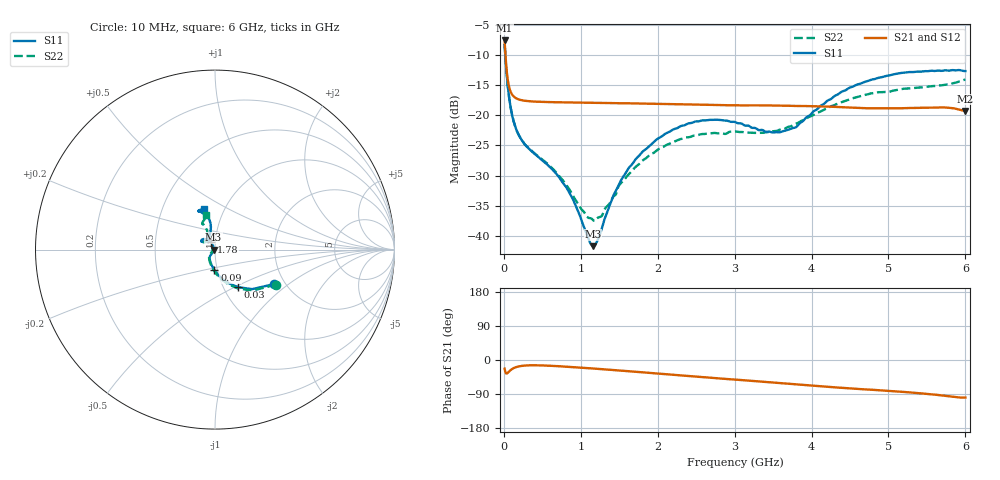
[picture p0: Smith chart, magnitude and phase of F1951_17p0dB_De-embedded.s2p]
! Integrated Device Technology
! Corporate Headquarters
! 6024 Silver Creek Valley Road
! San Jose, CA 95138  USA
! Phone:  1-408-284-8200
! Toll Free:  1-800-223-1366
! Webpage:  http://www.idt.com/
! Timing and RF Division
! 515 Groton Road, Suite 102
! Westford, MA 01886-6024
! Device:  F1951
! Description: 6-bit 0.5 dB Digital Step Attenuator
! Frequency:  100.0 -  4000.00 MHz
! Package:  4x4 mm Thin QFN Plastic Package: 24 pin
! Ports:  2 RF, 6 DC
!  Pin  1  = NC
!  Pin  2  = RF1  =  Port 1
!  Pin  3  = GND
!  Pin  4  = NC
!  Pin  5  = Serial Data Out (SDO)
!  Pin  6  = NC
!  Pin  7  = Reset Bar ( RSTb)
!  Pin  8  = Clock (CLK)
!  Pin  9  = Chip Select Bar (CSb)
!  Pin 10  = NC
!  Pin 11  = Serial Data In (SDI)
!  Pin 12  = NC
!  Pin 13  = NC
!  Pin 14  = VDD
!  Pin 15  = NC
!  Pin 16  = GND
!  Pin 17  = RF2  =  Port 2
!  Pin 18  = NC
!  Pin 19  = GND
!  Pin 20  = GND
!  Pin 21  = GND
!  Pin 22  = GND
!  Pin 23  = GND
!  Pin 24  = GND
! State:  34
! Atten State:  17.0 dB
! Voltage:  +3.30 Volts
! Current:  0.478 mA
! Data:  The device was measured on a F195X evaluation board which has
!  individual transmission lines to the RF pins.  Data was collected
!  de-embedded using a Automatic Fixture Removal [AFR] (Keysight Technologies).
!  The reference plane is the edge of the package pin.
! Misc:  Lot Code  1225BCA
!  Action Tracker AT0399
! Date Measured:  2018-09-13
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# GHz S dB R 50
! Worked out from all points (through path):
!   600 points, 10 MHz to 6 GHz, reference 50 ohm
!   highest |S21| = -7.60 dB at 10 MHz (marker M1); lowest = -19.3 dB at 6 GHz (marker M2)
!   group delay of S21, straight-line fit = 41 ps
!   lowest |S11| = -41.7 dB at 1.16 GHz (marker M3), VSWR 1.02, Z = 49.2 + j0.0511 ohm
!   |S11| at or under -10 dB: 18.05 MHz to end of sweep
!   |S22| runs from -37.5 to -8.2 dB; largest |S21 - S12| = 0.00027
!   S11 on the Smith chart (normalised r, x): 10 MHz: 1.76, -0.79; 30 MHz: 1.17, -0.52; 90 MHz: 0.97, -0.22; 1.78 GHz: 0.95, +0.08; 6 GHz: 0.80, +0.38
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0.01  -8.36 -30.2  -7.60 -23.0  -7.60 -23.0  -8.15 -30.0
0.03  -12.18 -58.3  -11.58 -35.5  -11.58 -35.6  -12.03 -59.7
0.06  -16.19 -79.2  -14.81 -32.1  -14.82 -32.1  -16.16 -81.2
0.09  -18.85 -91.4  -16.15 -26.3  -16.15 -26.3  -18.81 -93.8
0.16  -22.31 -108.7  -17.19 -18.8  -17.19 -18.8  -22.30 -111.2
0.25  -24.44 -119.6  -17.55 -15.1  -17.55 -15.1  -24.45 -123.0
0.71  -30.14 -127.4  -17.85 -16.3  -17.85 -16.4  -29.93 -137.2
0.87  -33.27 -129.2  -17.89 -18.5  -17.89 -18.5  -32.68 -142.1
1.01  -37.43 -138.3  -17.93 -20.4  -17.93 -20.4  -35.62 -152.1
1.16  -41.71 176.4  -17.95 -22.4  -17.95 -22.4  -37.40 -178.2
1.27  -38.96 134.5  -17.96 -24.1  -17.96 -24.1  -36.74 158.2
1.51  -31.14 115.9  -18.01 -27.7  -18.01 -27.7  -31.42 133.7
1.78  -26.39 118.7  -18.05 -32.2  -18.05 -32.2  -27.81 129.5
2.01  -23.82 125.4  -18.11 -35.9  -18.11 -35.9  -25.63 132.6
2.49  -21.03 138.9  -18.22 -43.7  -18.22 -43.7  -23.34 140.8
3.01  -21.15 149.2  -18.34 -51.9  -18.35 -51.8  -22.68 144.6
3.58  -22.84 128.7  -18.39 -60.8  -18.40 -60.8  -22.42 126.7
3.79  -22.03 112.8  -18.46 -64.2  -18.47 -64.1  -21.43 119.7
4.01  -19.56 103.5  -18.50 -67.6  -18.50 -67.6  -20.06 114.5
4.49  -15.46 100.5  -18.72 -74.9  -18.72 -74.8  -17.38 113.1
5.01  -13.40 108.8  -18.86 -81.5  -18.86 -81.5  -16.11 116.0
6  -12.67 105.8  -19.29 -99.1  -19.29 -99.1  -14.06 104.8
